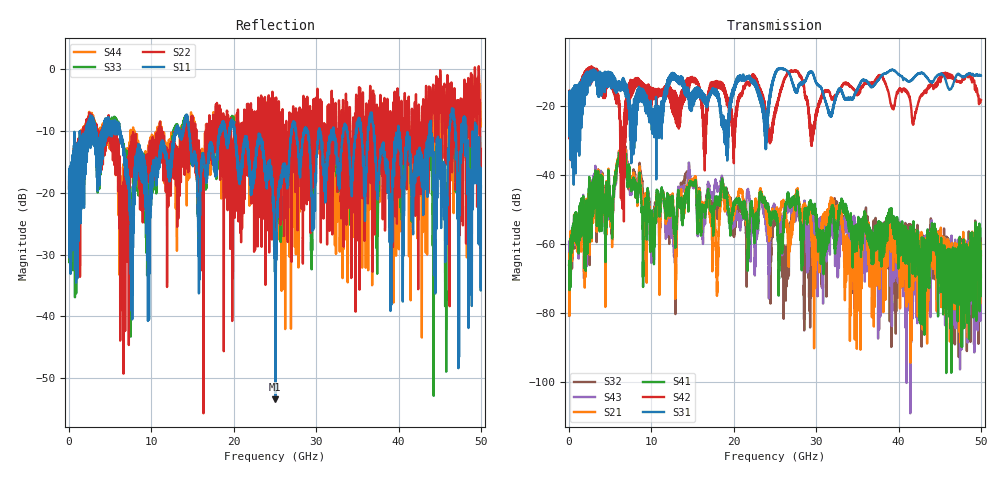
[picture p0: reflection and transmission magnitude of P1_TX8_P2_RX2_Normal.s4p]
!Keysight Technologies,N5225B,MY57041031,A.13.20.10
!Date: Friday, May 31, 2019 11:30:34
!Correction: S11(Full 4 Port(1,2,3,4))
!S12(Full 4 Port(1,2,3,4))
!S13(Full 4 Port(1,2,3,4))
!S14(Full 4 Port(1,2,3,4))
!S21(Full 4 Port(1,2,3,4))
!S22(Full 4 Port(1,2,3,4))
!S23(Full 4 Port(1,2,3,4))
!S24(Full 4 Port(1,2,3,4))
!S31(Full 4 Port(1,2,3,4))
!S32(Full 4 Port(1,2,3,4))
!S33(Full 4 Port(1,2,3,4))
!S34(Full 4 Port(1,2,3,4))
!S41(Full 4 Port(1,2,3,4))
!S42(Full 4 Port(1,2,3,4))
!S43(Full 4 Port(1,2,3,4))
!S44(Full 4 Port(1,2,3,4))
!S4P File: Measurements: <S11,S12,S13,S14>,
!<S21,S22,S23,S24>,
!<S31,S32,S33,S34>,
!<S41,S42,S43,S44>:
# Hz S  dB  R 50.0
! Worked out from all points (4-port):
!   5000 points, 10 MHz to 50 GHz, reference 50 ohm
!   strongest paths, dB at 10 MHz, 12.51 GHz, 25.01 GHz, 37.51 GHz, 50 GHz:
!     S31: -19.6, -10.8, -11.0, -12.6, -11.3
!     S42: -19.3, -15.9, -22.0, -11.5, -18.4
!     S41: -66.4, -47.6, -51.4, -57.3, -62.3
!     S21: -66.0, -47.7, -50.9, -64.9, -63.5
!     S43: -59.4, -51.9, -49.3, -69.1, -77.0
!     S32: -80.9, -52.5, -52.3, -64.8, -69.7
!   lowest |S11| = -53.3 dB at 25.05 GHz (marker M1), VSWR 1.00, Z = 49.8 - j0.0564 ohm
!   |S11| at or under -10 dB: 6.192 GHz to 12.89 GHz (6.696 GHz wide, 70.2 % of centre); 20.1 GHz to 26.99 GHz (6.89 GHz wide, 29.3 % of centre); 40 GHz to 43.76 GHz (3.761 GHz wide, 8.98 % of centre)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
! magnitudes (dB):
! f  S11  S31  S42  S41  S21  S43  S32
! 10 MHz  -19.4  -19.6  -19.3  -66.4  -66.0  -59.4  -80.9
! 6.74 GHz  -14.5  -13.9  -23.1  -39.9  -37.2  -38.4  -36.1
! 9.26 GHz  -15.7  -17.0  -14.7  -48.3  -45.5  -49.7  -53.2
! 25.05 GHz  -53.3  -10.5  -22.0  -50.8  -51.4  -49.9  -52.2
! 27.29 GHz  -8.5  -14.5  -9.9  -47.8  -52.3  -49.7  -50.6
! 29.52 GHz  -26.2  -10.4  -30.4  -50.2  -58.7  -51.3  -57.0
! 50 GHz  -22.9  -11.3  -18.4  -62.3  -63.5  -77.0  -69.7
